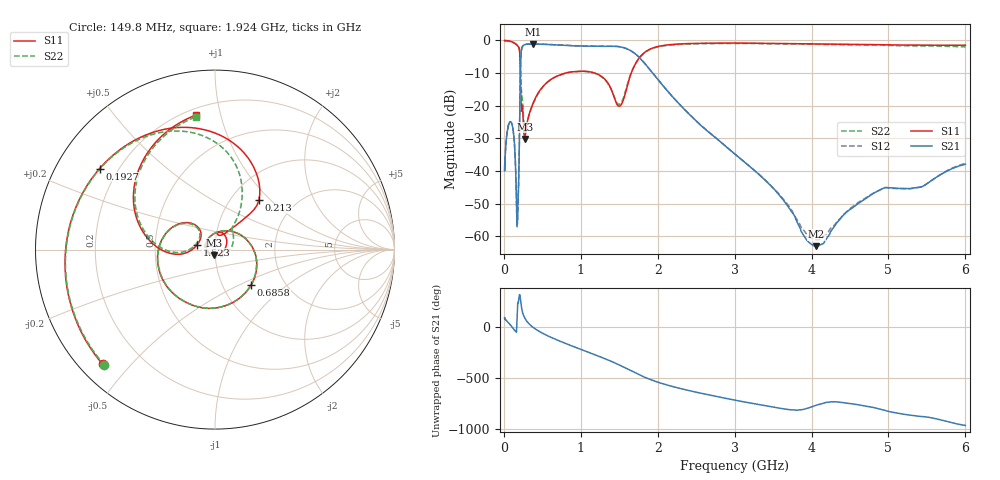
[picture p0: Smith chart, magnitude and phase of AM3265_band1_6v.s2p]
!Agilent Technologies,E8364B,MY43040894,A.07.50.67
!Agilent E8364B: A.07.50.67
!Date: Friday, May 09, 2025 07:16:29
!Correction: S11(Full 2 Port(1,2))
!S21(Full 2 Port(1,2))
!S12(Full 2 Port(1,2))
!S22(Full 2 Port(1,2))
!S2P File: Measurements: S11, S21, S12, S22:Log Frequency Sweep
# Hz S  dB  R 50
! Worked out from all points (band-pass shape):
!   3201 points, 10 MHz to 6 GHz, reference 50 ohm
!   highest |S21| = -1.09 dB at 378 MHz (marker M1); lowest = -63.0 dB at 4.063 GHz (marker M2)
!   |S21| within 3 dB of the highest: 223.9 MHz to 1.708 GHz (1.484 GHz wide, 154 % of centre)
!   lowest |S11| = -30.1 dB at 271.2 MHz (marker M3), VSWR 1.06, Z = 49.4 - j3.04 ohm
!   |S11| at or under -10 dB: 213.8 MHz to 802.3 MHz (588.6 MHz wide, 116 % of centre); 1.185 GHz to 1.656 GHz (470.6 MHz wide, 33.1 % of centre)
!   |S22| runs from -27.9 to -0.1 dB; largest |S21 - S12| = 0.0043
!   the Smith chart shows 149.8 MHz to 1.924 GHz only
!   S11 on the Smith chart (normalised r, x): 149.8 MHz: 0.07, -0.42; 192.7 MHz: 0.13, +0.31; 213 MHz: 1.34, +0.85; 685.8 MHz: 1.36, -0.59; 1.523 GHz: 0.82, +0.05; 1.924 GHz: 0.24, +0.84
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1e7  -0.05 -7.6  -39.62 94.9  -38.16 92.7  -0.09 -7.3
2.908064e7  -0.06 -21.6  -31.14 69.3  -31.05 69.2  -0.06 -21.6
8.439949e7  -0.25 -65.4  -24.87 23.2  -24.87 23.1  -0.28 -65.6
1.497977e8  -0.97 -134.5  -36.96 -38.9  -36.98 -40.3  -1.00 -133.7
1.722968e8  -1.45 -169.3  -56.42 92.9  -56.88 -72.2  -1.45 -167.4
1.927059e8  -2.10 144.9  -43.36 -91.2  -43.93 -90.9  -2.04 150.2
2.129627e8  -8.68 48.4  -12.41 -66.8  -12.38 -66.8  -6.48 75.1
2.44949e8  -21.33 41.3  -1.79 141.9  -1.75 141.8  -19.46 20.1
2.712392e8  -30.13 -98.9  -1.29 92.1  -1.25 92.1  -27.65 -95.3
3.779802e8  -19.36 71.5  -1.09 0.2  -1.06 0.1  -19.57 74.5
6.857793e8  -10.99 -44.7  -1.37 -123.4  -1.34 -123.4  -10.99 -45.1
7.123273e8  -10.72 -52.3  -1.41 -131.8  -1.37 -131.9  -10.73 -52.7
1.157832e9  -9.81 -172.0  -1.79 96.6  -1.76 96.6  -9.87 -172.9
1.522597e9  -19.76 164.5  -2.01 -19.4  -1.98 -19.4  -19.13 164.4
1.923806e9  -2.42 98.2  -9.67 -160.3  -9.64 -160.3  -2.52 98.0
2.067357e9  -1.56 62.8  -13.82 163.3  -13.79 163.3  -1.68 63.2
2.455151e9  -0.92 -11.0  -23.63 87.7  -23.60 87.7  -1.05 -10.4
2.96862e9  -0.79 -90.1  -34.08 7.0  -34.11 7.1  -0.90 -90.2
3.518433e9  -0.90 -166.5  -45.65 -69.3  -45.62 -68.5  -1.00 -168.3
4.063101e9  -1.07 122.2  -62.99 -48.3  -61.01 -175.4  -1.17 119.8
5.002045e9  -1.35 4.3  -45.09 -109.0  -45.20 -108.8  -1.53 4.8
6e9  -1.45 -115.1  -37.90 112.7  -37.62 112.7  -1.95 -110.9
